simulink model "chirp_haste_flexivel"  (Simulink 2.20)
settings: Solver=ode1  StartTime=0.0  StopTime=50  FixedStep=0.001  RelTol=1e-3  AbsTol=1e-6
libraries: winlib x4, simulink x1

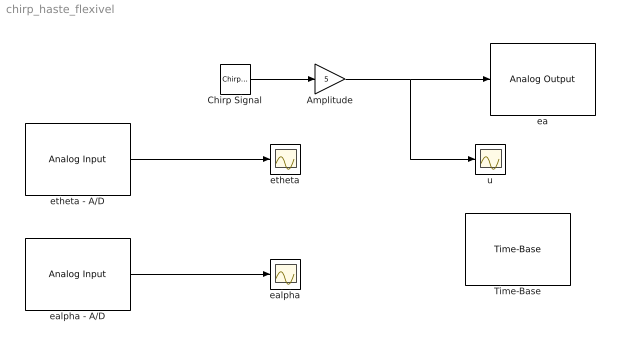
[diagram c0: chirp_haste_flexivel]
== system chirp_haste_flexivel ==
  Amplitude : Gain  Gain=5
  Chirp Signal : simulink/Sources/Chirp Signal  f1=0.1  T=10  f2=20
  Time-Base : winlib/Quanser Consulting MultiQ Series/Time-Base  baseAddr=0x320  irqLevel=9  clockSource=1
  ea : winlib/Quanser Consulting MultiQ Series/Analog Output  baseAddr=0x320  channels=[4]  initialOutputs=0  finalOutputs=0  sampleTime=str2num(get_param(bdroot, 'FixedStep'))
  ealpha : Scope
  ealpha - A/D : winlib/Quanser Consulting MultiQ Series/Analog Input  baseAddr=0x320  channels=[2]  sampleTime=str2num(get_param(bdroot, 'FixedStep'))
  etheta : Scope
  etheta - A/D : winlib/Quanser Consulting MultiQ Series/Analog Input  baseAddr=0x320  channels=[1]  sampleTime=str2num(get_param(bdroot, 'FixedStep'))
  u : Scope
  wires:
  etheta - A/D/1 -> etheta/1
  Chirp Signal/1 -> Amplitude/1
  Amplitude/1 -> ea/1, u/1
  ealpha - A/D/1 -> ealpha/1
